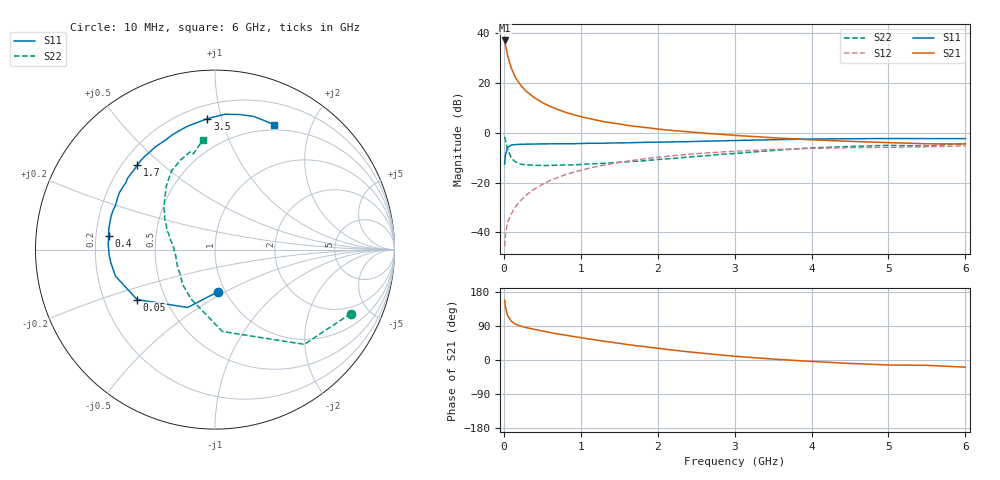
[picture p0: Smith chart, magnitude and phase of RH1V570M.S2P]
! SIEMENS Small Signal Semiconductors
! BFR106
! Si NPN RF Bipolar Junction Transistor in SOT23
! VCE = 1.5 V  IC = 70 mA
! Common Emitter S-Parameters:  August  1996
# GHz  S  MA  R  50
!  f  S11  S21  S12  S22
! GHz  MAG  ANG  MAG  ANG  MAG  ANG  MAG  ANG
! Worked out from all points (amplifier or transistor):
!   36 points, 10 MHz to 6 GHz, reference 50 ohm
!   highest |S21| = 37.2 dB at 10 MHz (marker M1)
!   |S21| within 3 dB of that: start of sweep to 29.43 MHz
!   unconditionally stable (mu >= 1): 174.6 MHz to 3.388 GHz; 4.251 GHz to end of sweep
!   at 250 MHz: K = 1.07, MAG = 20.6 dB, |S12| = -26.2 dB
!   at 1.4 GHz: K = 1.07, MAG = 6.5 dB, |S12| = -12.4 dB
!   at 6 GHz: K = 1.02, MAG = -0.5 dB, |S12| = -5.2 dB
!   S11 on the Smith chart (normalised r, x): 10 MHz: 0.93, -0.46; 50 MHz: 0.34, -0.26; 400 MHz: 0.25, +0.06; 1.7 GHz: 0.26, +0.41; 3.5 GHz: 0.29, +0.90; 6 GHz: 0.44, +1.49
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0.01  0.235 -85.8  72.29 158.1  0.0053 75.7  0.8365 -25.2
0.02  0.3566 -115.3  60.67 141.6  0.0092 67.3  0.7254 -46.7
0.05  0.5155 -147.3  35.32 116.3  0.0162 57.4  0.4584 -84.8
0.1  0.5741 -165.1  19.45 101.7  0.0241 62.5  0.3054 -116.1
0.15  0.5847 -172.8  13.19 94.9  0.0326 66.4  0.2645 -133.4
0.2  0.59 -176.6  10.02 90.7  0.0409 69.2  0.2398 -143.3
0.25  0.5927 179.7  8.004 87.4  0.0491 70.7  0.2315 -151.6
0.3  0.5961 177.5  6.707 85.1  0.058 71.6  0.2287 -156.4
0.4  0.5976 172.7  5.078 80.7  0.0751 72.0  0.2236 -164.2
0.5  0.6029 169.2  4.084 76.6  0.0927 71.5  0.2214 -169.4
0.6  0.605 165.4  3.422 72.6  0.1104 70.4  0.222 -172.7
0.7  0.6083 162.0  2.962 68.8  0.1273 69.3  0.2254 -175.7
0.9  0.6068 155.9  2.342 62.2  0.1614 66.1  0.2282 178.3
1.1  0.6199 149.3  1.958 55.7  0.1938 62.9  0.238 174.7
1.3  0.6214 143.2  1.691 49.7  0.2255 59.3  0.2454 170.1
1.7  0.6391 132.6  1.36 38.3  0.2842 52.3  0.2691 162.3
2.2  0.6621 120.0  1.117 26.1  0.3494 43.3  0.3068 152.6
2.8  0.6925 106.5  0.944 13.7  0.4114 32.9  0.3686 140.5
3.5  0.7309 93.3  0.8 2.4  0.4658 21.8  0.4442 127.8
4.5  0.7651 79.6  0.678 -9.1  0.5037 7.8  0.5351 111.0
5.5  0.7693 68.3  0.606 -14.1  0.5263 -0.6  0.5473 102.7
6  0.7697 64.6  0.6 -18.9  0.551 -7.2  0.6163 96.1
